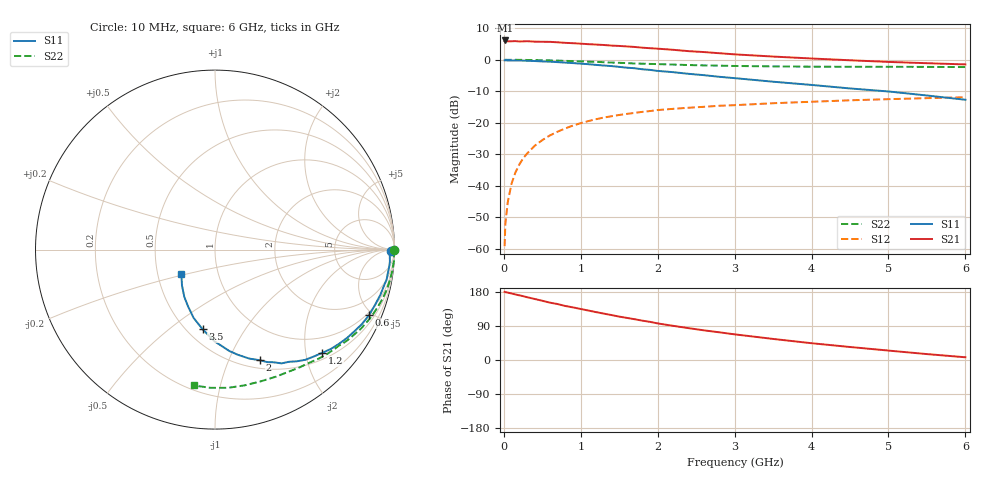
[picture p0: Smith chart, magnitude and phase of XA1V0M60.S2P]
! SIEMENS Discrete & RF Semiconductors
! BFY180
! Si NPN RF Bipolar Junction Transistor in MICRO-X
! VCE = 1 V  IC = 0.6 mA
! Common Emitter S-Parameters:  May  1997
# GHz  S  MA  R  50
!  f  S11  S21  S12  S22
! GHz  MAG  ANG  MAG  ANG  MAG  ANG  MAG  ANG
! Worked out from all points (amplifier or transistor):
!   36 points, 10 MHz to 6 GHz, reference 50 ohm
!   highest |S21| = 6.1 dB at 20 MHz (marker M1)
!   |S21| within 3 dB of that: start of sweep to 2.216 GHz
!   unconditionally stable (mu >= 1): 3.976 GHz to end of sweep
!   at 250 MHz: K = 0.06, MSG = 18.6 dB, |S12| = -31.3 dB
!   at 1.4 GHz: K = 0.47, MSG = 11.2 dB, |S12| = -17.9 dB
!   at 6 GHz: K = 1.08, MAG = 3.5 dB, |S12| = -11.9 dB
!   S11 on the Smith chart (normalised r, x): 10 MHz: 85, -20; 600 MHz: 0.85, -4.75; 1.2 GHz: 0.63, -2.33; 2 GHz: 0.59, -1.31; 3.5 GHz: 0.60, -0.66; 6 GHz: 0.66, -0.19
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0.01  0.9779 -0.3  1.959 179.9  0.0011 92.2  0.9983 -0.2
0.02  0.9808 -0.8  2.026 179.0  0.0025 83.1  0.9999 -0.6
0.05  0.9744 -1.8  1.963 177.9  0.0054 83.8  0.9978 -1.2
0.1  0.9767 -4.0  1.965 175.5  0.0108 86.8  0.9976 -2.5
0.15  0.9748 -6.0  1.979 173.1  0.0162 86.4  0.9988 -3.8
0.2  0.9722 -7.6  1.953 170.7  0.0216 83.8  0.9964 -5.0
0.3  0.9643 -11.6  1.971 165.8  0.0322 81.1  0.9929 -7.5
0.4  0.955 -15.4  1.941 161.1  0.043 78.8  0.9891 -10.0
0.6  0.9324 -23.1  1.925 151.3  0.0631 72.7  0.9773 -14.8
0.8  0.9006 -30.3  1.857 142.5  0.0816 67.0  0.9608 -19.6
1.1  0.8504 -40.6  1.768 130.5  0.1064 59.2  0.9341 -26.2
1.2  0.8291 -44.0  1.744 126.3  0.1141 56.6  0.9257 -28.3
1.5  0.7714 -53.8  1.658 114.5  0.133 50.1  0.8945 -34.3
2  0.6655 -67.9  1.501 96.5  0.1592 41.2  0.8538 -42.9
2.2  0.6361 -72.6  1.44 90.2  0.1664 37.7  0.8392 -46.3
2.6  0.5702 -82.0  1.326 78.3  0.1792 32.6  0.8139 -52.1
2.8  0.5369 -86.2  1.271 73.1  0.1861 30.2  0.8066 -54.9
3.5  0.4487 -98.9  1.125 55.6  0.2043 22.9  0.7854 -64.2
4  0.3987 -107.4  1.048 44.3  0.2157 17.9  0.777 -70.9
4.5  0.3507 -115.3  0.982 34.3  0.2273 13.3  0.7742 -77.7
5.5  0.271 -132.8  0.882 15.6  0.2459 4.5  0.7706 -91.8
6  0.2321 -143.7  0.844 7.2  0.2544 -0.3  0.7661 -98.8
